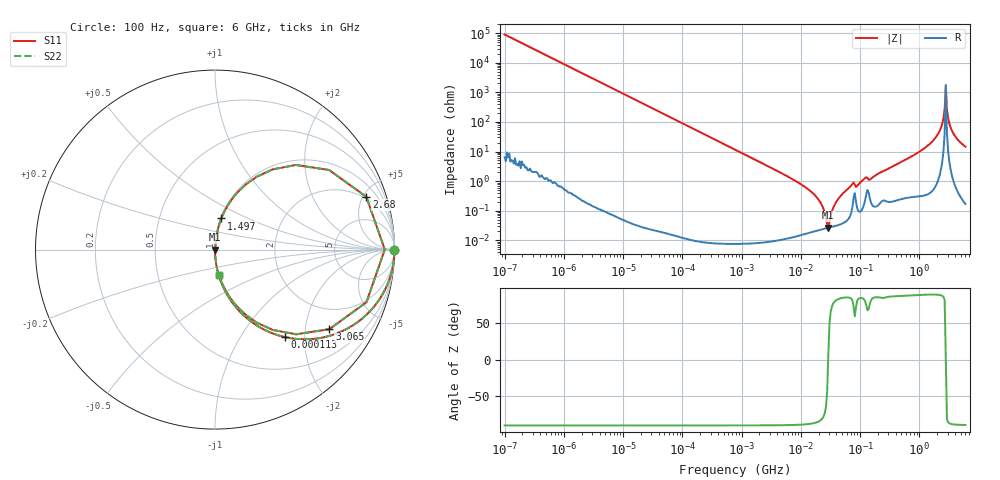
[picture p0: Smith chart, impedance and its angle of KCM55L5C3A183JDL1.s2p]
!Murata Part Number: KCM55L5C3A183JDL1
!These Parameters are Measured in Series Mode Connection
!Data Generated on Mar 13, 2026
!  o--ll--o
!Port1  Port2
!  o------o
!Operation Temp=25[degC], DC Bias Voltage=0[V]
!Freq. Start=100[Hz] Stop=6[GHz] 401[Steps]
# Hz S RI R 50
!Freq.(Hz) S11(Real) S11(Imag) S21(Real) S21(Imag) S12(Real) S12(Imag) S22(Real) S22(Imag)
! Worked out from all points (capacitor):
!   401 points, 100 Hz to 6 GHz, reference 50 ohm
!   read as one part in series: C = 17.6 nF near 109 Hz
!   lowest |Z| = 26.6 mohm at 29.12 MHz (marker M1)
!   series resonance near 28.98 MHz, so ESL is about 1.7 nH
!   S11 on the Smith chart (normalised r, x): 100 Hz: open; 113 kHz: 1.00, -1.60; 1.497 GHz: 1.01, +0.36; 2.68 GHz: 1.82, +5.29; 3.065 GHz: 1.21, -2.70; 6 GHz: 1.00, -0.29
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100  1 -0.00111  1.3e-06 0.00111  1.3e-06 0.00111  1 -0.00111
2008  0.9995 -0.0222  0.000494 0.0222  0.000494 0.0222  0.9995 -0.0222
11009  0.9854 -0.1199  0.0146 0.1199  0.0146 0.1199  0.9854 -0.1199
40335  0.8341 -0.3719  0.1659 0.3719  0.1659 0.3719  0.8341 -0.3719
112960  0.3908 -0.4879  0.6092 0.4879  0.6092 0.4879  0.3908 -0.4879
252896  0.1135 -0.3171  0.8865 0.3171  0.8865 0.3171  0.1135 -0.3171
774597  0.0135 -0.1151  0.9865 0.1151  0.9865 0.1151  0.0135 -0.1151
6644369  0.000286 -0.0128  0.9997 0.0128  0.9997 0.0128  0.000286 -0.0128
1.555665e7  0.000209 -0.0041  0.9998 0.0041  0.9998 0.0041  0.000209 -0.0041
2.128304e7  0.00023 -0.00193  0.9998 0.00193  0.9998 0.00193  0.00023 -0.00193
2.911731e7  0.000264 2.93e-05  0.9997 -2.93e-05  0.9997 -2.93e-05  0.000264 2.93e-05
3.983537e7  0.000316 0.00201  0.9997 -0.00201  0.9997 -0.00201  0.000316 0.00201
7.129496e7  0.000936 0.00719  0.9991 -0.00719  0.9991 -0.00719  0.000936 0.00719
3.124326e8  0.00272 0.0274  0.9973 -0.0274  0.9973 -0.0274  0.00272 0.0274
1.497423e9  0.0352 0.1737  0.9648 -0.1737  0.9648 -0.1737  0.0352 0.1737
2.240541e9  0.2315 0.4053  0.7685 -0.4053  0.7685 -0.4053  0.2315 0.4053
2.450438e9  0.4502 0.4717  0.5498 -0.4717  0.5498 -0.4717  0.4502 0.4717
2.679998e9  0.8431 0.2941  0.1569 -0.2941  0.1569 -0.2941  0.8431 0.2941
3.065283e9  0.6371 -0.4433  0.3629 0.4433  0.3629 0.4433  0.6371 -0.4433
3.352442e9  0.3206 -0.4472  0.6794 0.4472  0.6794 0.4472  0.3206 -0.4472
3.8344e9  0.1337 -0.3286  0.8663 0.3286  0.8663 0.3286  0.1337 -0.3286
6e9  0.0225 -0.1426  0.9775 0.1426  0.9775 0.1426  0.0225 -0.1426
